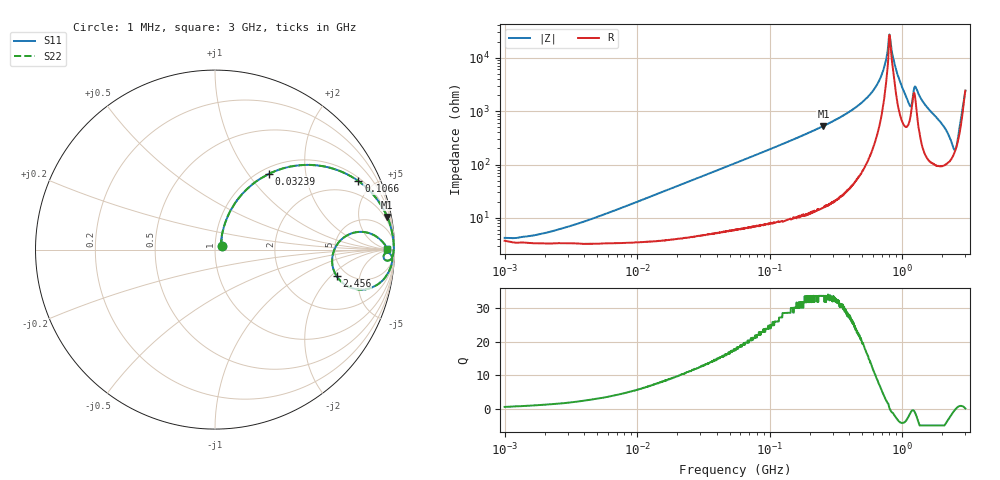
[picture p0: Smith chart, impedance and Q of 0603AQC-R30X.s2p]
!s-Parameter Generated by FASTRON Sdn. Bhd.
!FASTRON P/N : 0603AQC-R30X
!Keysight Technologies: E4991B_MY54100416_A.01.15
!Date: Thu Jun 25 14:07:22 2026
!Version  :Rev00  Thu Jun 25 14:07:22 2026
!Data & Calibration Information:
!Freq  S11  S21  S12  S22
!PortZ  Port1:50+j0  Port2:50+j0
!When reading reference impedance value at option line is always used.
! Remarks : This data is being provided solely for informational purposes.
# Hz S dB R 50
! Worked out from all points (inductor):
!   1601 points, 1 MHz to 3 GHz, reference 50 ohm
!   read as one part in series: L = 315 nH near 4.984 MHz
!   highest Q = 33.7 at 254.5 MHz (marker M1), where L = 328 nH
!   self-resonance near 800.6 MHz
!   S11 on the Smith chart (normalised r, x): 1 MHz: 1.07, +0.04; 32.39 MHz: 1.10, +1.26; 106.6 MHz: 1.17, +4.11; 2.456 GHz: 4.13, -2.35; 3 GHz: 49, +3
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1000000  -27.80 27.1  -0.32 -1.1  -0.32 -1.1  -27.80 27.1
3804036  -22.00 62.3  -0.30 -4.2  -0.30 -4.2  -22.00 62.3
1.447069e7  -11.50 67.2  -0.63 -15.3  -0.63 -15.3  -11.50 67.2
3.238729e7  -5.75 54.7  -1.74 -30.9  -1.74 -30.9  -5.75 54.7
5.504702e7  -3.00 41.8  -3.51 -45.0  -3.51 -45.0  -3.00 41.8
1.065605e8  -1.06 25.5  -7.30 -62.2  -7.30 -62.2  -1.06 25.5
2.083556e8  -0.30 13.4  -12.70 -74.9  -12.70 -74.9  -0.30 13.4
2.545267e8  -0.20 10.7  -14.60 -77.6  -14.60 -77.6  -0.20 10.7
4.219165e8  -0.07 5.3  -20.60 -82.4  -20.60 -82.4  -0.07 5.3
5.840965e8  -0.04 2.6  -26.80 -83.1  -26.80 -83.1  -0.04 2.6
7.064253e8  -0.03 1.1  -34.10 -77.8  -34.10 -77.8  -0.03 1.1
7.925923e8  -0.03 0.2  -47.30 -42.1  -47.30 -42.1  -0.03 0.2
8.208471e8  -0.04 -0.2  -45.30 32.6  -45.30 32.6  -0.04 -0.2
9.302341e8  -0.05 -1.2  -33.10 72.9  -33.10 72.9  -0.05 -1.2
1.125055e9  -0.29 -3.6  -23.10 60.7  -23.10 60.7  -0.29 -3.6
1.274982e9  -0.15 -1.9  -28.70 61.1  -28.70 61.1  -0.15 -1.9
1.481494e9  -0.10 -4.2  -22.60 79.0  -22.60 79.0  -0.10 -4.2
2.040726e9  -0.42 -10.1  -14.90 69.6  -14.90 69.6  -0.42 -10.1
2.312676e9  -1.41 -15.2  -10.90 51.1  -10.90 51.1  -1.41 -15.2
2.455801e9  -3.18 -12.3  -9.00 24.6  -9.00 24.6  -3.18 -12.3
2.634014e9  -2.23 6.9  -12.00 -21.8  -12.00 -21.8  -2.23 6.9
3e9  -0.35 0.2  -28.00 -3.6  -28.00 -3.6  -0.35 0.2
